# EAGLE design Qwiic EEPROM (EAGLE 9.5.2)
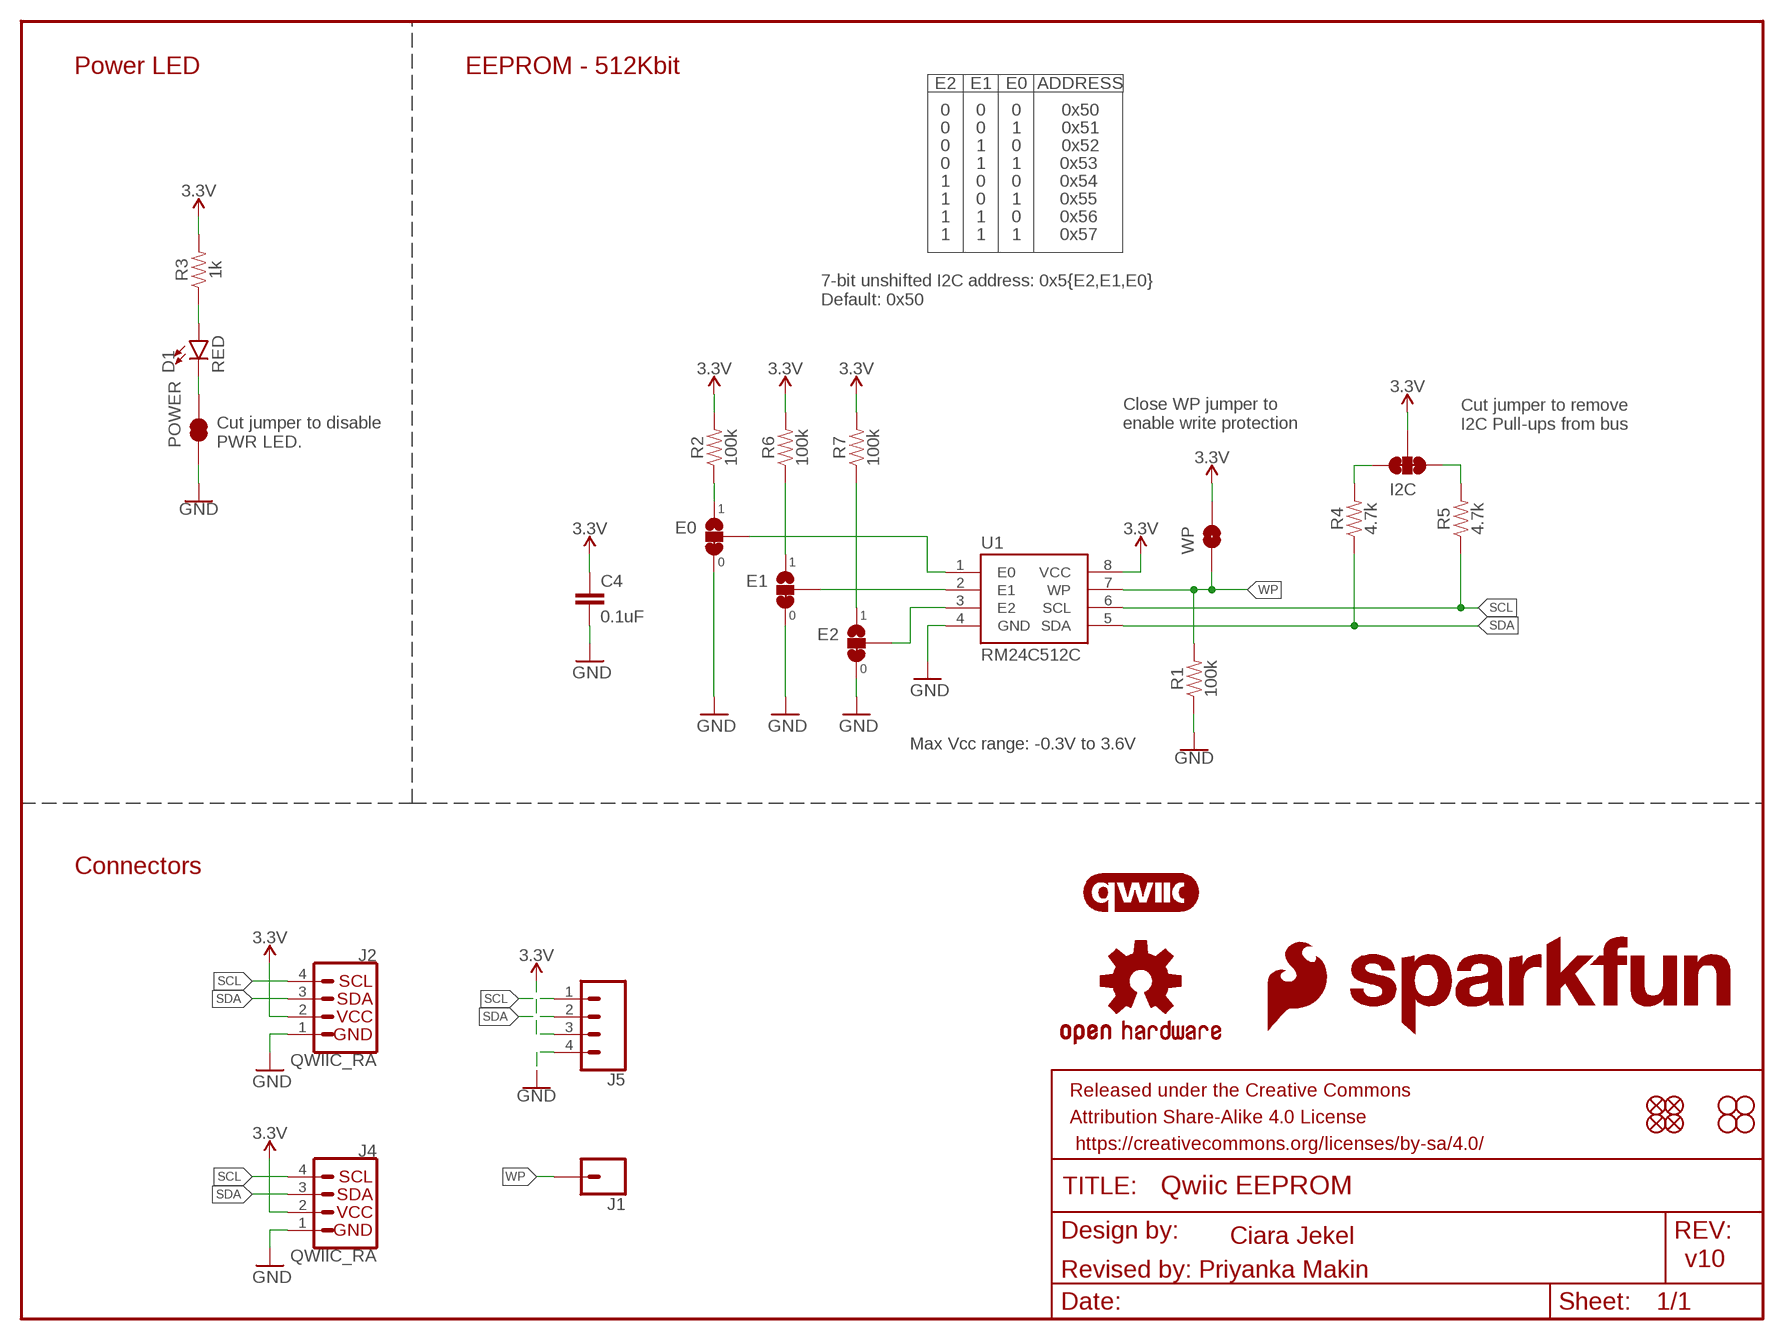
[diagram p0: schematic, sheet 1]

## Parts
C4  0.1uF  0.1UF-0603-25V-(+80/-20%)  [0603]
D1  RED  LED-RED0603  [LED-0603]
E0  JUMPER-SMT_3_1-NC_TRACE_SILK  [SMT-JUMPER_3_1-NC_TRACE_SILK]
E1  JUMPER-SMT_3_1-NC_TRACE_SILK  [SMT-JUMPER_3_1-NC_TRACE_SILK]
E2  JUMPER-SMT_3_1-NC_TRACE_SILK  [SMT-JUMPER_3_1-NC_TRACE_SILK]
FRAME1  FRAME-LETTER  [CREATIVE_COMMONS]
I2C  JUMPER-SMT_3_2-NC_TRACE_SILK  [SMT-JUMPER_3_2-NC_TRACE_SILK]
J1  CONN_01PTH_NO_SILK_YES_STOP  [1X01_NO_SILK]
J2  QWIIC_RA  QWIIC_CONNECTORJS-1MM  [JST04_1MM_RA]
J4  QWIIC_RA  QWIIC_CONNECTORJS-1MM  [JST04_1MM_RA]
J5  CONN_041X04_NO_SILK_NO_POP  [1X04_NO_SILK]
JP1  FIDUCIALUFIDUCIAL  [FIDUCIAL-MICRO]
JP2  FIDUCIALUFIDUCIAL  [FIDUCIAL-MICRO]
JP3  STAND-OFF  [STAND-OFF]
JP4  STAND-OFF  [STAND-OFF]
JP5  FIDUCIALUFIDUCIAL  [FIDUCIAL-MICRO]
JP6  FIDUCIALUFIDUCIAL  [FIDUCIAL-MICRO]
JP7  STAND-OFF  [STAND-OFF]
JP8  STAND-OFF  [STAND-OFF]
LOGO1  OSHW-LOGOMINI  [OSHW-LOGO-MINI]
LOGO2  SFE_LOGO_NAME.1_INCH  [SFE_LOGO_NAME_.1]
LOGO3  SFE_LOGO_FLAME.1_INCH  [SFE_LOGO_FLAME_.1]
LOGO4  QWIIC_LOGO_4MM  [QWIIC_4MM]
POWER  JUMPER-SMT_2_NC_TRACE_SILK  [SMT-JUMPER_2_NC_TRACE_SILK]
R1  100k  100KOHM-0603-1/10W-1%  [0603]
R2  100k  100KOHM-0603-1/10W-1%  [0603]
R3  1k  1KOHM-0603-1/10W-1%  [0603]
R4  4.7k  4.7KOHM-0603-1/10W-1%  [0603]
R5  4.7k  4.7KOHM-0603-1/10W-1%  [0603]
R6  100k  100KOHM-0603-1/10W-1%  [0603]
R7  100k  100KOHM-0603-1/10W-1%  [0603]
U1  RM24C512C  [SO08]
WP  JUMPER-SMT_2_NO_SILK  [SMT-JUMPER_2_NO_SILK]

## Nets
3.3V: C4.1 I2C.2 J2.2 J4.2 J5.3 R2.2 R3.2 R6.2 R7.2 U1.8(VCC) WP.2
GND: C4.2 E0.3 E1.3 E2.3 J2.1 J4.1 J5.4 POWER.1 R1.1 U1.4(GND)
N$1: I2C.1 R5.2
N$2: I2C.3 R4.2
N$3: D1.A R3.1
N$4: E2.2 U1.3(E2)
N$5: E1.2 U1.2(E1)
N$6: E0.2 U1.1(E0)
N$7: E0.1 R2.1
N$8: E2.1 R7.1
N$9: E1.1 R6.1
N$10: D1.C POWER.2
SCL: J2.4 J4.4 J5.1 R5.1 U1.6(SCL)
SDA: J2.3 J4.3 J5.2 R4.1 U1.5(SDA)
WP: J1.1 R1.2 U1.7(WP) WP.1

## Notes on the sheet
- Power LED | EEPROM - 512Kbit
- E2 | E1 | E0 | ADDRESS
- 0 | 0 | 0 | 0x50
- 0 | 0 | 1 | 0x51
- 0 | 1 | 0 | 0x52
- 0 | 1 | 1 | 0x53
- 1 | 0 | 0 | 0x54
- 1 | 0 | 1 | 0x55
- 1 | 1 | 0 | 0x56
- 1 | 1 | 1 | 0x57
- 7-bit unshifted I2C address: 0x5{E2,E1,E0}
  Default: 0x50
- Cut jumper to remove 
  I2C Pull-ups from bus
- Cut jumper to disable 
  PWR LED.
- Close WP jumper to 
  enable write protection
- 1
- 0 | 1
- 0 | 1
- 0
- Max Vcc range: -0.3V to 3.6V
- Connectors
- Ciara Jekel
- v10
- Revised by: Priyanka Makin

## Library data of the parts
C4 = SparkFun-Capacitors:0.1UF: 0.1µF ceramic capacitors; PROD_ID: CAP-00810
D1 = SparkFun-LED:LED-RED: Red SMD LED; PROD_ID: DIO-00819
E0 E1 E2 = SparkFun-Jumpers:JUMPER-SMT_3_1-NC_TRACE: Normally closed trace jumper (1 of 2 connections) This jumper has a trace between two pads so it's normally closed (NC). The other connection is normally open (NO). Use a razor knife to open the connection. For best results follow the IPC guidelines for cutting traces: Cutout at least 0.063 mm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
FRAME1 = SparkFun-Aesthetics:FRAME-LETTER: Schematic Frame - Letter
I2C = SparkFun-Jumpers:JUMPER-SMT_3_2-NC_TRACE: Normally closed trace jumper (2 of 2 connections) This jumper has a trace between all three pads so they are normally closed (NC). Use a razor knife to open the connection(s). For best results follow the IPC guidelines for cutting traces: Cutout at least 0.063 mm (0.005 in). Remove all loose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
J1 = SparkFun-Connectors:CONN_01: Single connection point. Often used as Generic Header-pin footprint for 0.1 inch spaced/style header connections
J2 J4 = SparkFun-Connectors:QWIIC_CONNECTOR: SparkFun I2C Standard Qwiic Connector An SMD 1mm pitch JST connector makes it easy and quick (get it? Qwiic?) to connect I2C devices to each other. The Qwiic system enables fast and solderless connection between popular platforms and various sensors and actuators. We carry 200mm, 100mm, 50mm, and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; PROD_ID: CONN-13694; VALUE: QWIIC_RIGHT_ANGLE
J5 = SparkFun-Connectors:CONN_04: Multi connection point. Often used as Generic Header-pin footprint for 0.1 inch spaced/style header connections On any of the 0.1 inch spaced packages, you can populate with these: Break Away Headers - Straight (PRT-00116) Break Away Male Headers - Right Angle (PRT-00553) Female Headers (PRT-00115)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
JP1 JP2 JP5 JP6 = SparkFun-Aesthetics:FIDUCIAL: Fiducial Alignment Points
JP3 JP4 JP7 JP8 = SparkFun-Hardware:STAND-OFF: Stand Off
LOGO1 = SparkFun-Aesthetics:OSHW-LOGO: Open-Source Hardware (OSHW) Logo
LOGO2 = SparkFun-Aesthetics:SFE_LOGO_NAME: SparkFun Font Logo
LOGO3 = SparkFun-Aesthetics:SFE_LOGO_FLAME: SparkFun Flame Logo
LOGO4 = SparkFun-Aesthetics:QWIIC_LOGO: Qwiic Logos for placement on schematic and PCB. The 5.5mm silk logo is best for placing next to Qwiic connector.
POWER = SparkFun-Jumpers:JUMPER-SMT_2_NC_TRACE: Normally closed trace jumper
R1 R2 R6 R7 = SparkFun-Resistors:100KOHM: 100kΩ resistor; PROD_ID: RES-07828
R3 = SparkFun-Resistors:1KOHM: 1kΩ resistor; PROD_ID: RES-07856
R4 R5 = SparkFun-Resistors:4.7KOHM: 4.7kΩ resistor; PROD_ID: RES-07857
U1 = SparkFun-IC-Memory:RM24C512C; PROD_ID: IC-14645
WP = SparkFun-Jumpers:JUMPER-SMT_2_NO: Normally open jumper

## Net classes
1 power: width 0.203 mm

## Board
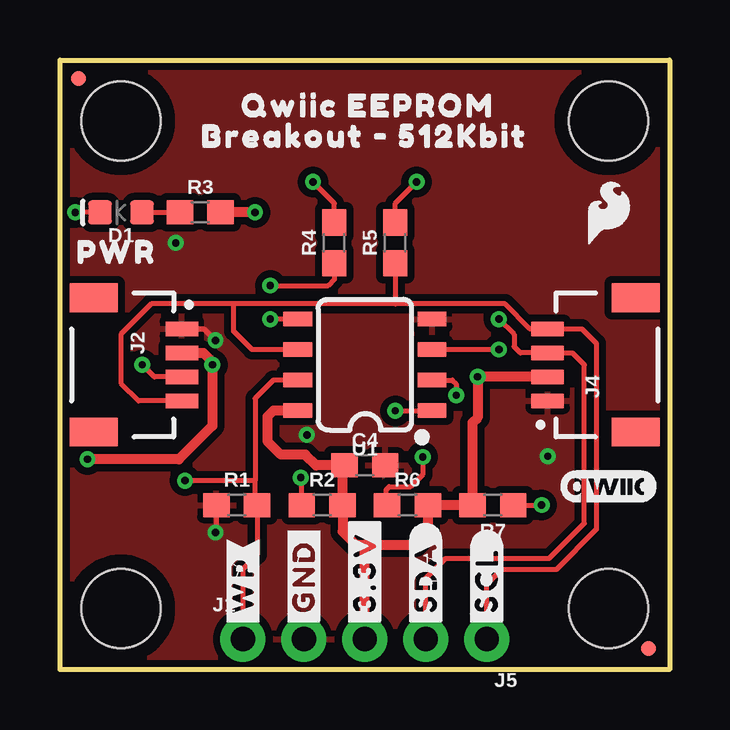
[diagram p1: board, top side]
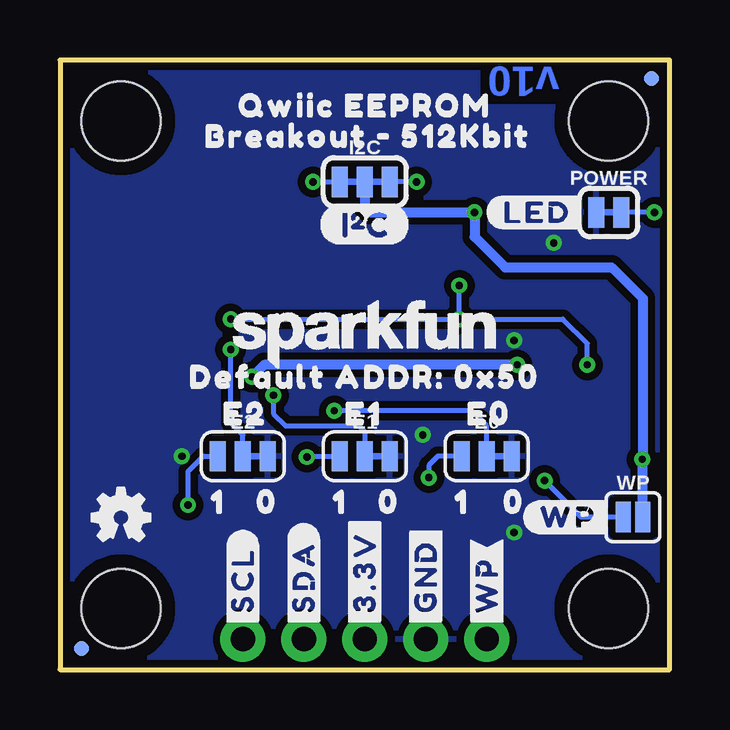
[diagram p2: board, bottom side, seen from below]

Size 25.4 x 25.4 mm. Coordinates in mm from the lower left corner, seen from the top.
Outline: 0,0 0,25.4 25.4,25.4 25.4,0 0,0
Copper layers (1*16): Top 0.035mm / dielectric 1.5mm / Bottom 0.035mm
Design rules "SparkFun-2-Layer-General-JLCPCB": minimum track width 7mil, minimum drill 0.3mm, track to track 7mil, track to pad 7mil, pad to pad 7mil, via to via 7mil, smd to smd 7mil, copper to edge 7mil, drill to drill 7mil, minimum pad ring 7mil, minimum via ring 7mil, stop-mask expansion 3mil, vias tented up to drill 25mil, thermal gap 10mil

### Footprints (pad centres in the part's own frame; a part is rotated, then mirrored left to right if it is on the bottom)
0603 = smd 1.1 x 1: 1 -0.85,0; 2 0.85,0
LED-0603 = smd 1 x 1: A -0.877,0; C 0.877,0
SMT-JUMPER_3_1-NC_TRACE_SILK = smd 0.66 x 1.27: 1 -1.041,0; 2 0,0; 3 1.041,0
SMT-JUMPER_3_2-NC_TRACE_SILK = smd 0.66 x 1.27: 1 -1.041,0; 2 0,0; 3 1.041,0
1X01_NO_SILK = drill 1.016 pad 1.88: 1 0,0
JST04_1MM_RA = smd 0.6 x 1.35: 1 -1.5,0; 2 -0.5,0; 3 0.5,0; 4 1.5,0 | smd 1.2 x 2: NC1 2.8,-3.675; NC2 -2.8,-3.675
1X04_NO_SILK = drill 1.016 pad 1.88: 1 0,0; 2 2.54,0; 3 5.08,0; 4 7.62,0
FIDUCIAL-MICRO = smd 0.635 x 0.635: 1 0,0
STAND-OFF = hole 3.302: 0,0
SMT-JUMPER_2_NC_TRACE_SILK = smd 0.66 x 1.27: 1 -0.521,0; 2 0.521,0
SO08 = smd 0.6 x 1.2: 1 -1.905,-2.8; 2 -0.635,-2.8; 3 0.635,-2.8; 4 1.905,-2.8; 5 1.905,2.8; 6 0.635,2.8; 7 -0.635,2.8; 8 -1.905,2.8
SMT-JUMPER_2_NO_SILK = smd 0.635 x 1.27: 1 -0.406,0; 2 0.406,0

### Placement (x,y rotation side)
C4  12.7,8.51 0 top
D1  2.54,19.05 180 top
E0  7.62,8.89 0 bottom
E1  12.7,8.89 0 bottom
E2  17.78,8.89 0 bottom
FRAME1  not placed on the board
I2C  12.7,20.32 0 bottom
J1  7.62,1.27 0 top
J2  5.08,12.7 270 top
J4  20.32,12.7 90 top
J5  17.78,1.27 180 top
JP1  0.76,24.64 0 bottom
JP2  24.51,0.89 0 top
JP3  2.54,22.86 0 top
JP4  22.86,22.86 0 top
JP5  24.51,0.89 0 bottom
JP6  0.76,24.64 0 top
JP7  2.54,2.54 0 top
JP8  22.86,2.54 0 top
LOGO1  22.86,6.35 0 bottom
LOGO2  12.7,13.97 0 bottom
LOGO3  22.86,19.05 0 top
LOGO4  22.86,7.62 0 top
POWER  2.54,19.05 0 bottom
R1  7.37,6.86 0 top
R2  10.92,6.86 0 top
R3  5.84,19.05 0 top
R4  11.43,17.78 90 top
R5  13.97,17.78 90 top
R6  14.48,6.86 0 top
R7  18.03,6.86 180 top
U1  12.7,12.7 90 top
U$1  [#WP#3]  7.62,1.65 90 top
U$2  [#WP#3]  7.62,1.65 90 bottom
U$3  [#WP#0]  6.1,6.35 0 bottom
U$4  [E00]  9.14,10.67 0 bottom
U$5  [E10]  14.22,10.67 0 bottom
U$6  [E20]  19.3,10.67 0 bottom
U$7  [00]  7.62,6.99 0 bottom
U$8  [00]  12.83,6.99 0 bottom
U$9  [00]  17.91,6.99 0 bottom
U$10  [#GND#0]  10.16,1.65 90 top
U$11  [(I_SUPER2_C)]  14.61,18.54 0 bottom
U$12  [PWR0]  0,17.4 0 top
U$13  [10]  19.81,6.99 0 bottom
U$14  [#GND#0]  10.16,1.65 90 bottom
U$15  [#3#3V#0]  12.7,1.65 90 top
U$16  [#3#3V#0]  12.7,1.65 90 bottom
U$17  [#SDA#0]  15.24,1.65 90 top
U$18  [#LED#2]  7.62,19.05 0 bottom
U$19  [QWIIC_EEPROM0]  6.86,23.5 0 top
U$20  [QWIIC_EEPROM0]  18.67,23.5 0 bottom
U$21  [10]  14.73,6.99 0 bottom
U$22  [10]  9.65,6.99 0 bottom
U$23  [BREAKOUT_#_512KBIT0]  5.21,22.23 0 top
U$24  [BREAKOUT_#_512KBIT0]  20.07,22.23 0 bottom
U$25  [DEFAULT_ADDR#_0X500]  20.7,12.19 0 bottom
U$29  [#SDA#0]  15.24,1.65 90 bottom
U$30  [#SCL#0]  17.78,1.65 90 top
U$31  [#SCL#0]  17.78,1.65 90 bottom
WP  1.52,6.35 0 bottom

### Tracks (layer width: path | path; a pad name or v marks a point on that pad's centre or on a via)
3.3V  (via drill 0.3)
  Top 0.203: 6.35,12.83 v6.35,12.7 | 11.77,8.43 C4.1
  Top 0.406: J2.2 5.98,13.2 6.35,12.83 | v6.35,12.7 6.35,10.16 4.95,8.76 v1.14,8.76 | C4.1 10.67,8.51 10.22,8.95 9.21,8.95 8.64,9.53 8.64,10.54 8.89,10.79 U1.8 | 12.7,5.21 12.32,5.21 11.77,5.75 R2.2 11.77,8.43 | 12.7,5.21 14.82,5.21 15.33,5.71 R6.2 R7.2 17.18,10.29 17.4,10.5 v17.4,12.2 J4.2 | J5.3 12.7,5.21 | v8.13,19.05 R3.2
  Bottom 0.203: v1.14,8.76 1.12,8.76
  Bottom 0.406: WP.2 1.12,8.76 1.12,15.47 2.41,16.76 6.86,16.76 8.13,18.03 v8.13,19.05 12.45,19.05 12.7,19.3 I2C.2 | v6.35,12.7 16.9,12.7 v17.4,12.2
GND  (via drill 0.3)
  Top 0.203: J2.1 5.99,14.2 v6.48,13.72 | R1.1 6.52,5.75 v6.48,5.71
  other vias: 20.32,8.89 4.83,17.78 10.29,9.78
  pour Bottom (isolate 0.305): 0,0 0,25.4 25.4,25.4 25.4,0
  pour Top (isolate 0.305): 0,0 0,25.4 25.4,25.4 25.4,0
N$1  (via drill 0.3)
  Top 0.203: R5.2 13.97,19.43 v14.86,20.32
  Bottom 0.203: v14.86,20.32 I2C.1
N$2  (via drill 0.3)
  Top 0.203: R4.2 11.43,19.43 v10.54,20.32
  Bottom 0.203: v10.54,20.32 I2C.3
N$3
  Top 0.203: D1.A R3.1
N$4  (via drill 0.3)
  Top 0.203: v18.29,13.34 U1.3
  Bottom 0.203: E2.2 17.78,9.78 18.29,10.29 v18.29,13.34
N$5  (via drill 0.3)
  Top 0.203: U1.2 16.35,12.06 16.51,11.9 v16.51,11.43
  Bottom 0.203: v16.51,11.43 16.51,10.67 16,10.16 12.95,10.16 12.7,9.91 E1.2
N$6  (via drill 0.3)
  Top 0.203: v13.97,10.78 15.49,10.78 U1.1
  Bottom 0.203: E0.2 7.62,10.16 8.26,10.79 13.96,10.79 v13.97,10.78
N$7  (via drill 0.3)
  Top 0.203: R2.1 10.07,7.96 v10.03,8
  Bottom 0.203: E0.1 9.65,8.89 10.03,8.51 v10.03,8
N$8  (via drill 0.3)
  Top 0.203: R7.1 v20.07,6.86
  Bottom 0.203: v20.07,6.86 20.07,8.26 19.43,8.89 E2.1
N$9  (via drill 0.3)
  Top 0.203: R6.1 13.59,6.9 13.59,7.49 13.72,7.62 14.61,7.62 15.11,8.13 v15.11,8.86
  Bottom 0.203: E1.1 15.08,8.89 v15.11,8.86
N$10  (via drill 0.3)
  Top 0.203: D1.C v0.64,19.05
  Bottom 0.203: v0.64,19.05 POWER.2
SCL
  Top 0.203: 13.97,15.24 18.54,15.24 19.58,14.2 J4.4 21.74,14.2 22.35,13.59 22.35,5.84 20.7,4.19 18.41,4.19 17.78,3.56 J5.1 | 13.97,15.24 7.24,15.24 | 7.24,15.24 3.81,15.24 2.54,13.97 2.54,11.94 3.28,11.2 J2.4 | U1.6 8,13.34 7.24,14.1 7.24,15.24 | R5.1 13.97,15.24
SDA  (via drill 0.3)
  Top 0.203: v18.29,14.61 18.92,13.97 18.92,13.46 19.18,13.2 J4.3 21.34,13.2 21.84,12.7 21.84,6.1 20.38,4.64 16.07,4.64 15.24,3.81 J5.2 | J2.3 3.93,12.2 v3.43,12.7 | U1.5 v8.76,14.61 | R4.1 11.43,16.26 11.18,16 v8.76,16
  Bottom 0.203: v3.43,12.7 3.43,13.59 4.45,14.61 v8.76,14.61 | v18.29,14.61 v8.76,14.61 | v8.76,14.61 v8.76,16
WP  (via drill 0.3)
  Top 0.203: U1.7 8.89,12.06 8.13,11.3 8.13,7.87 | J1.1 7.62,4.19 8.22,4.79 R1.2 8.13,6.95 8.13,7.87 | 8.13,7.87 v5.21,7.87
  Bottom 0.203: WP.1 3.68,6.35 v5.21,7.87

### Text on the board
Bottom: v10
Measures: Dimensions in Inches
tDocu: Ciara Jekel | Revised by: Priyanka Makin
